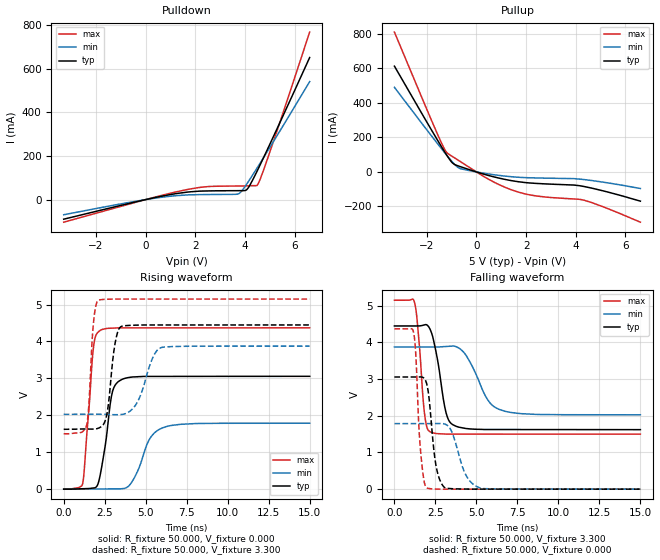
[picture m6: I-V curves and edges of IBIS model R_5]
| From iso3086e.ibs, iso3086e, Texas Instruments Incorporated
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|   R_5 MODEL
[Model]   R_5
Model_type   3-state
Polarity   Non-Inverting
Enable   Active-Low
Vmeas   = 2.59
Cref   = 15pF
|   typ   min   max
C_comp   3.47pF   4.23pF   3.64pF
|C_comp (High state)   1.69pF   1.71pF   1.69pF
[Voltage Range]   5   4.5   5.5
[Temperature Range]   40   125   -40
[Pullup Reference]   5   4.5   5.5
[Pulldown Reference]   0   0   0
[Power Clamp Reference]   5   4.5   5.5
[GND Clamp Reference]   0   0   0
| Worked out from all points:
|   slope of the pulldown table from 0 to 0.75 V, typ, clamps not added: 41.7 ohm
|   slope of the pullup table from 0 to 0.75 V, typ, clamps not added: 24.7 ohm
|   falling waveform, R_fixture 50.000, V_fixture 3.300: 20-80 % time 625ps typ, 1.2ns min, 373ps max; typ from 4.45 V to 1.62 V
|   rising waveform, R_fixture 50.000, V_fixture 0.000: 20-80 % time 566ps typ, 979ps min, 429ps max; typ from 0.001 V to 3.06 V
|   rising waveform, R_fixture 50.000, V_fixture 3.300: 20-80 % time 419ps typ, 841ps min, 273ps max; typ from 1.62 V to 4.45 V
|   falling waveform, R_fixture 50.000, V_fixture 0.000: 20-80 % time 430ps typ, 782ps min, 305ps max; typ from 3.06 V to 0.001 V
[Pulldown]
|   Voltage   I(typ)   I(min)   I(max)
-3.3V     -89.75mA   -69.39mA   -103.5mA
-706.2mV  -18.6mA    -13.69mA   -21.89mA
1.11V     25.36mA    16.83mA    32.32mA
2.293V    39.16mA    22.99mA    57.43mA
3.689V    40.88mA    24.87mA    62.26mA
3.843V    40.94mA    36.33mA    62.32mA
4.066V    45.45mA    71.14mA    62.81mA
4.229V    73.22mA    99.34mA    63.87mA
4.471V    127.5mA    142.6mA    64.22mA
4.605V    159mA      166.9mA    92.85mA
4.912V    232.9mA    223.2mA    189.8mA
6.6V      650.9mA    540.4mA    767.3mA
[Pullup]
|   Voltage   I(typ)   I(min)   I(max)
-3.3V     612.5mA    489.8mA    809.7mA
-1.567V   184.4mA    164.2mA    218.9mA
-1.29V    118.8mA    113.8mA    133.6mA
-1.147V   86.6mA     88.26mA    106.2mA
-889.3mV  43.81mA    45.41mA    82.24mA
-646.8mV  30.64mA    19.06mA    59.99mA
432.3mV   -18.4mA    -10.42mA   -37.74mA
1.442V    -51.19mA   -28.14mA   -105.1mA
2.407V    -66.45mA   -34.81mA   -139.1mA
4.323V    -84.18mA   -44.06mA   -163.5mA
5.165V    -111.8mA   -60.55mA   -205.4mA
6.6V      -169.1mA   -95.93mA   -291mA
[Ramp]
R_load = 50
|   typ   min   max
dV/dt_r   1.29384/5.65785e-010  0.908858/9.79654e-010   1.74337/4.28854e-010
dV/dt_f   1.0206/6.23606e-010  0.675573/1.19616e-009   1.263/3.72554e-010
[Falling Waveform]
R_fixture = 50.000
V_fixture = 3.300
V_fixture_min = 3.150
V_fixture_max = 3.600
C_fixture = 0.000
|  time   V(typ)   V(min)   V(max)
0s        4.448V     3.875V     5.149V
1.233ns   4.448V     3.875V     5.077V
1.386ns   4.448V     3.875V     4.599V
1.827ns   4.476V     3.875V     2.089V
2.173ns   4.358V     3.875V     1.565V
2.599ns   3.598V     3.875V     1.514V
3.136ns   2.105V     3.888V     1.501V
3.74ns    1.718V     3.887V     1.501V
6.417ns   1.626V     2.17V      1.501V
15ns      1.622V     2.027V     1.5V
[Rising Waveform]
R_fixture = 50.000
V_fixture = 0.000
V_fixture_min = 0.000
V_fixture_max = 0.000
C_fixture = 0.000
|  time   V(typ)   V(min)   V(max)
0s        588uV      905.5uV    263.8uV
1.166ns   11.85mV    3.694mV    173.5mV
1.827ns   33.03mV    5.274mV    3.886V
2.225ns   382.2mV    6.225mV    4.301V
2.983ns   2.657V     8.038mV    4.362V
3.553ns   2.973V     13.16mV    4.369V
4.139ns   3.035V     182mV      4.369V
5.193ns   3.054V     1.324V     4.369V
5.977ns   3.054V     1.652V     4.369V
15ns      3.057V     1.786V     4.37V
[Rising Waveform]
R_fixture = 50.000
V_fixture = 3.300
V_fixture_min = 3.150
V_fixture_max = 3.600
C_fixture = 0.000
|  time   V(typ)   V(min)   V(max)
0s        1.622V     2.027V     1.5V
1.386ns   1.63V      2.029V     1.711V
1.535ns   1.628V     2.029V     2.288V
1.827ns   1.628V     2.029V     4.558V
2.12ns    1.653V     2.03V      5.118V
2.599ns   1.96V      2.025V     5.144V
3.136ns   3.957V     2.017V     5.149V
3.553ns   4.415V     2.024V     5.149V
5.977ns   4.447V     3.839V     5.149V
15ns      4.448V     3.875V     5.149V
[Falling Waveform]
R_fixture = 50.000
V_fixture = 0.000
V_fixture_min = 0.000
V_fixture_max = 0.000
C_fixture = 0.000
|  time   V(typ)   V(min)   V(max)
0s        3.057V     1.786V     4.37V
1.166ns   3.057V     1.786V     4.276V
1.287ns   3.057V     1.786V     3.791V
1.599ns   3.059V     1.786V     1.021V
1.987ns   2.835V     1.786V     32.88mV
2.533ns   647mV      1.788V     3.584mV
3.06ns    44.3mV     1.776V     471.3uV
4.373ns   3.521mV    372.9mV    448.5uV
5.193ns   1.777mV    37.48mV    434.2uV
15ns      588uV      905.5uV    263.8uV
